|   IBIS file stm32l496_4a6_wlcsp100.ibs
[IBIS ver]   4.2
[File name]   stm32l496_4a6_wlcsp100.ibs
[File Rev]   4.0
[Date]   08-10-2018
[Source]   Data Created at STMicroelectronics
[Notes]   File originated from ELDO simulations.
[Disclaimer]  This information is for modeling purpose only and is
   not guaranteed.
   The information is subject to change without notice.
[Copyright]   Copyright 2018 STMicroelectronics Inc.
|   Component stm32l496_4a6_wlcsp100
[Component] stm32l496_4a6_wlcsp100
[Manufacturer] STMicroelectronics
[Package]
| variable   typ   min   max
R_pkg   0.0   0.0   0.0
L_pkg   0.0H   0.0H   0.0H
C_pkg   0.0F   0.0F   0.0F
[Pin]  signal_name   model_name   R_pin   L_pin   C_pin
A1 VDDUSB POWER
A10 VDD POWER
A2 PA15 io8prog2m25m50m120m_sudq_ft
A3 PD1 io8prog2m25m50m120m_sudq_ft
A4 VDD POWER
A5 PG10 io8prog2m25m50m120m_sudq_ft
A6 VDDIO2 POWER
A7 PB6 io8prog2m25m50m120m_sudq_i2c_ft
A8 PB9 io8prog2m25m50m120m_sudq_i2c_ft
A9 VSS GND
B1 VSS GND
B10 PE3 io8prog2m25m50m120m_sudq_ft
B2 PA14 io8prog2m25m50m120m_sudq_ft
B3 PD0 io8prog2m25m50m120m_sudq_ft
B4 PD4 io8prog2m25m50m120m_sudq_ft
B5 PG9 io8prog2m25m50m120m_sudq_ft
B6 PG12 io8prog2m25m50m120m_sudq_ft
B7 PB5 io8prog2m25m50m120m_sudq_ft
B8 PB8 io8prog2m25m50m120m_sudq_i2c_ft
B9 PE2 io8prog2m25m50m120m_sudq_ft
C1 PA12 io8usblsfs_otg2
C10 VBAT POWER
C2 PA13 io8prog2m25m50m120m_sudq_ft
C3 PC11 io8prog2m25m50m120m_sudq_ft
C4 PC12 io8prog2m25m50m120m_sudq_ft
C5 PD7 io8prog2m25m50m120m_sudq_ft
C6 PB3 io8prog2m25m50m120m_sudq_ft
C7 PB4 io8prog2m25m50m120m_sudq_i2c_ft
C8 PE4 io8prog2m25m50m120m_sudq_ft
C9 PC13 io8prog2m25m50m120m_sudq_ft
D1 PA11 io8usblsfs_otg2
D2 PA10 io8usb_id_otg20_lcd4_ft_ms
D3 PA9 POWER
D4 PC10 io8prog2m25m50m120m_sudq_ft
D5 PD6 io8prog2m25m50m120m_sudq_ft
D6 PG11 io8prog2m25m50m120m_sudq_ft
D7 PB7 io8prog2m25m50m120m_sudq_i2c_ft
D8 PE5 io8prog2m25m50m120m_sudq_ft
D9 VSS GND
D10 PC14-OSC32_IN io8prog2m25m50m120m_sudq_ft
E1 PC8 io8prog2m25m50m120m_sudq_ft
E2 PC9 io8prog2m25m50m120m_sudq_i2c_ft
E3 PA8 io8w_swp_lcd4_ft
E4 PD2 io8prog2m25m50m120m_sudq_ft
E5 PD5 io8prog2m25m50m120m_sudq_ft
E6 PH3-BOOT0 io8prog2m25m50m120m_sudq_ft
E7 PE6 io8prog2m25m50m120m_sudq_ft
E8 NRST ioreset_ft_v33
E9 VDD POWER
E10 PC15-OSC32_OUT io8prog2m25m50m120m_sudq_ft
F1 VDD POWER
F2 PC6 io8prog2m25m50m120m_sudq_ft
F3 PC7 io8prog2m25m50m120m_sudq_ft
F4 PD15 io8prog2m25m50m120m_sudq_ft
F5 PB2 io8prog2m25m50m120m_sudq_ft
F6 PA4 io8prog2m25m50m120m_sudq_ft
F7 PC3 io8prog2m25m50m120m_sudq_ft
F8 PC1 io8prog2m25m50m120m_sudq_i2c_ft
F9 PC0 io8prog2m25m50m120m_sudq_i2c_ft
F10 PH0-OSC_IN io8prog2m25m50m120m_sudq_ft
G1 PD10 io8prog2m25m50m120m_sudq_ft
G10 PH1-OSC_OUT io8prog2m25m50m120m_sudq_ft
G2 PD9 io8prog2m25m50m120m_sudq_ft
G3 PD14 io8prog2m25m50m120m_sudq_ft
G4 PE13 io8prog2m25m50m120m_sudq_ft
G5 PE12 io8prog2m25m50m120m_sudq_ft
G6 PA5 io8prog2m25m50m120m_sudq_ft
G7 VREF+ POWER
G8 VREF- GND
G9 PA0 io8prog2m25m50m120m_sudq_ft
H1 PB15 io8prog2m25m50m120m_sudq_ft
H10 PC2 io8prog2m25m50m120m_sudq_ft
H2 PB14 io8prog2m25m50m120m_sudq_i2c_ft
H3 PD8 io8prog2m25m50m120m_sudq_ft
H4 PE15 io8prog2m25m50m120m_sudq_ft
H5 PE10 io8prog2m25m50m120m_sudq_ft
H6 PC4 io8prog2m25m50m120m_sudq_ft
H7 PA2 io8prog2m25m50m120m_sudq_ft
H8 PA1 io8prog2m25m50m120m_sudq_ft
H9 VSSA GND
J1 PB12 io8w_swp_lcd4_ft
J10 VDDA POWER
J2 PB13 io8prog2m25m50m120m_sudq_i2c_ft
J3 PB11 io8prog2m25m50m120m_sudq_i2c_ft
J4 PE14 io8prog2m25m50m120m_sudq_ft
J5 PE9 io8prog2m25m50m120m_sudq_ft
J6 PB0 io8prog2m25m50m120m_sudq_ft
J7 PA7 io8prog2m25m50m120m_sudq_i2c_ft
J8 VDD POWER
J9 PA3 io8prog2m25m50m120m_sudq_ft
K1 VDD POWER
K10 VSS GND
K2 VSS GND
K3 PB10 io8prog2m25m50m120m_sudq_i2c_ft
K4 PE11 io8prog2m25m50m120m_sudq_ft
K5 PE8 io8prog2m25m50m120m_sudq_ft
K6 PE7 io8prog2m25m50m120m_sudq_ft
K7 PB1 io8prog2m25m50m120m_sudq_ft
K8 PC5 io8prog2m25m50m120m_sudq_ft
K9 PA6 io8prog2m25m50m120m_sudq_ft
[Diff Pin]   inv_pin   vdiff   tdelay_typ  tdelay_min  tdelay_max
C1 D1 200mV   NA   NA   NA
[Model Selector] io8usblsfs_otg2
usb_ls_pd  "USB Low Speed mode - Pull Down"
usb_ls_pu2  "USB Low Speed mode - Pull up 2"
usb_ls_pu  "USB Low Speed mode - Pull up"
usb_fs  "USB Low Speed mode"
usb_fs_pd  "USB Full Speed mode - Pull Down"
usb_fs_pu2  "USB Full Speed mode - Pull up 2"
usb_fs_pu  "USB Full Speed mode - Pull up"
[Model Selector] io8usb_id_otg20_lcd4_ft_ms
io8usbid_1v8_id_pu  "ID 1V8 range with pull up"
io8usbid_3v3_id_pu  "ID 3V3 range with pull up"
io8usbid_1v8_id  "ID 1V8 range"
io8usbid_3v3_id  "ID 3V3 range"
io8lsusbid_1v8_pd  "GPIO 1.8V range with pd io low speed"
io8lsusbid_1v8_pu  "GPIO 1.8V range with pu io low speed"
io8lsusbid_1v8  "GPIO 1.8V range io low speed"
io8lsusbid_3v3_pd  "GPIO 3.3V range with pd io low speed"
io8lsusbid_3v3_pu  "GPIO 3.3V range with pu io low speed"
io8lsusbid_3v3  "GPIO 3.3V range io low speed"
io8fsusbid_1v8_pd  "GPIO 1.8V range with pd io full speed"
io8fsusbid_1v8_pu  "GPIO 1.8V range with pu io full speed"
io8fsusbid_1v8  "GPIO 1.8V range io full speed"
io8fsusbid_3v3_pd  "GPIO 3.3V range with pd io full speed"
io8fsusbid_3v3_pu  "GPIO 3.3V range with pu io full speed"
io8fsusbid_3v3  "GPIO 3.3V range io full speed"
io8msusbid_1v8_pd  "GPIO 1.8V range with pd io medium speed"
io8msusbid_1v8_pu  "GPIO 1.8V range with pu io medium speed"
io8msusbid_1v8  "GPIO 1.8V range io medium speed"
io8msusbid_3v3_pd  "GPIO 3.3V range with pd io medium speed"
io8msusbid_3v3_pu  "GPIO 3.3V range with pu io medium speed"
io8msusbid_3v3  "GPIO 3.3V range io medium speed"
io8hsusbid_1v8_pd  "GPIO 1.8V range with pd io high speed"
io8hsusbid_1v8_pu  "GPIO 1.8V range with pu io high speed"
io8hsusbid_1v8  "GPIO 1.8V range io high speed"
io8hsusbid_3v3_pd  "GPIO 3.3V range with pd io high speed"
io8hsusbid_3v3_pu  "GPIO 3.3V range with pu io high speed"
io8hsusbid_3v3  "GPIO 3.3V range io high speed"
[Model Selector] io8w_swp_lcd4_ft
io8w_swp_classc  "Class C swp functionality"
io8w_swp_classb  "Class B swp functionality"
io8lsw_1v8_pd  "GPIO 1.8V range with pd io low speed"
io8lsw_1v8_pu  "GPIO 1.8V range with pu io low speed"
io8lsw_1v8  "GPIO 1.8V range io low speed"
io8lsw_3v3_pd  "GPIO 3.3V range with pd io low speed"
io8lsw_3v3_pu  "GPIO 3.3V range with pu io low speed"
io8lsw_3v3  "GPIO 3.3V range io low speed"
io8fsw_1v8_pd  "GPIO 1.8V range with pd io full speed"
io8fsw_1v8_pu  "GPIO 1.8V range with pu io full speed"
io8fsw_1v8  "GPIO 1.8V range io full speed"
io8fsw_3v3_pd  "GPIO 3.3V range with pd io full speed"
io8fsw_3v3_pu  "GPIO 3.3V range with pu io full speed"
io8fsw_3v3  "GPIO 3.3V range io full speed"
io8msw_1v8_pd  "GPIO 1.8V range with pd io medium speed"
io8msw_1v8_pu  "GPIO 1.8V range with pu io medium speed"
io8msw_1v8  "GPIO 1.8V range io medium speed"
io8msw_3v3_pd  "GPIO 3.3V range with pd io medium speed"
io8msw_3v3_pu  "GPIO 3.3V range with pu io medium speed"
io8msw_3v3  "GPIO 3.3V range io medium speed"
io8hsw_1v8_pd  "GPIO 1.8V range with pd io high speed"
io8hsw_1v8_pu  "GPIO 1.8V range with pu io high speed"
io8hsw_1v8  "GPIO 1.8V range io high speed"
io8hsw_3v3_pd  "GPIO 3.3V range with pd io high speed"
io8hsw_3v3_pu  "GPIO 3.3V range with pu io high speed"
io8hsw_3v3  "GPIO 3.3V range io high speed"
[Model Selector] io8prog2m25m50m120m_sudq_ft
iols8p_sudq_ft_pd_lv  "IO low speed, PD=40kOhm - 1P8V"
iols8p_sudq_ft_pu_lv  "IO low speed, PU=40kOhm - 1P8V"
iols8p_sudq_ft_lv  "IO low speed - 1P8V"
iols8p_sudq_ft_pd  "IO low speed, PD=40kOhm - 3P3V"
iols8p_sudq_ft_pu  "IO low speed, PU=40kOhm - 3P3V"
iols8p_sudq_ft  "IO low speed - 3P3V"
iofs8p_sudq_ft_pd_lv  "IO full speed, PD=40kOhm - 1P8V"
iofs8p_sudq_ft_pu_lv  "IO full speed, PU=40kOhm - 1P8V"
iofs8p_sudq_ft_lv  "IO full speed - 1P8V"
iofs8p_sudq_ft_pd  "IO full speed, PD=40kOhm - 3P3V"
iofs8p_sudq_ft_pu  "IO full speed, PU=40kOhm - 3P3V"
iofs8p_sudq_ft  "IO full speed - 3P3V"
ioms8p_sudq_ft_pd_lv  "IO medium speed, PD=40kOhm - 1P8V"
ioms8p_sudq_ft_pu_lv  "IO medium speed, PU=40kOhm - 1P8V"
ioms8p_sudq_ft_lv  "IO medium speed - 1P8V"
ioms8p_sudq_ft_pd  "IO medium speed, PD=40kOhm - 3P3V"
ioms8p_sudq_ft_pu  "IO medium speed, PU=40kOhm - 3P3V"
ioms8p_sudq_ft  "IO medium speed - 3P3V"
iohs8p_sudq_ft_pd_lv  "IO high speed, PD=40kOhm - 1P8V"
iohs8p_sudq_ft_pu_lv  "IO high speed, PU=40kOhm - 1P8V"
iohs8p_sudq_ft_lv  "IO high speed - 1P8V"
iohs8p_sudq_ft_pd  "IO high speed, PD=40kOhm - 3P3V"
iohs8p_sudq_ft_pu  "IO high speed, PU=40kOhm - 3P3V"
iohs8p_sudq_ft  "IO high speed - 3P3V"
[Model Selector] io8prog2m25m50m120m_sudq_i2c_ft
io8prog_1v8_i2c_pd  "5V Tol GPIO 1.8V range i2c functionality with pull down"
io8prog_1v8_i2c_pu  "5V Tol GPIO 1.8V range i2c functionality with pull up"
io8prog_1v8_i2c  "5V Tol GPIO 1.8V range i2c functionality"
io8prog_3v3_i2c_pd  "5V Tol GPIO 3.3V range i2c functionality with pull down"
io8prog_3v3_i2c_pu  "5V Tol GPIO 3.3V range i2c functionality with pull up"
io8prog_3v3_i2c  "5V Tol GPIO 3.3V range i2c functionality"
io8ls_1v8_pd  "5V Tol GPIO 1.8V range with pd io low speed"
io8ls_1v8_pu  "5V Tol GPIO 1.8V range with pu io low speed"
io8ls_1v8  "5V Tol GPIO 1.8V range io low speed"
io8ls_3v3_pd  "5V Tol GPIO 3.3V range with pd io low speed"
io8ls_3v3_pu  "5V Tol GPIO 3.3V range with pu io low speed"
io8ls_3v3  "5V Tol GPIO 3.3V range io low speed"
io8fs_1v8_pd  "5V Tol GPIO 1.8V range with pd io full speed"
io8fs_1v8_pu  "5V Tol GPIO 1.8V range with pu io full speed"
io8fs_1v8  "5V Tol GPIO 1.8V range io full speed"
io8fs_3v3_pd  "5V Tol GPIO 3.3V range with pd io full speed"
io8fs_3v3_pu  "5V Tol GPIO 3.3V range with pu io full speed"
io8fs_3v3  "5V Tol GPIO 3.3V range io full speed"
io8ms_1v8_pd  "5V Tol GPIO 1.8V range with pd io medium speed"
io8ms_1v8_pu  "5V Tol GPIO 1.8V range with pu io medium speed"
io8ms_1v8  "5V Tol GPIO 1.8V range io medium speed"
io8ms_3v3_pd  "5V Tol GPIO 3.3V range with pd io medium speed"
io8ms_3v3_pu  "5V Tol GPIO 3.3V range with pu io medium speed"
io8ms_3v3  "5V Tol GPIO 3.3V range io medium speed"
io8hs_1v8_pd  "5V Tol GPIO 1.8V range with pd io high speed"
io8hs_1v8_pu  "5V Tol GPIO 1.8V range with pu io high speed"
io8hs_1v8  "5V Tol GPIO 1.8V range io high speed"
io8hs_3v3_pd  "5V Tol GPIO 3.3V range with pd io high speed"
io8hs_3v3_pu  "5V Tol GPIO 3.3V range with pu io high speed"
io8hs_3v3  "5V Tol GPIO 3.3V range io high speed"
[Model Selector] ioreset_ft_v33
ioreset_1v2_pu  "RESET 1.2V range with PU"
ioreset_1v2  "RESET 1.2V range"
ioreset_1v8_pu  "RESET 1.8V range with PU"
ioreset_1v8  "RESET 1.8V range"
ioreset_3v3_pu  "RESET 3.3V range with PU"
ioreset_3v3  "RESET 3.3V range"
| Models and submodels in the file (121): usb_ls_pd (I/O), usb_ls_pu2 (I/O), usb_ls_pu (I/O), usb_fs (I/O), usb_fs_pd (I/O), usb_fs_pu2 (I/O), usb_fs_pu (I/O), io8usbid_1v8_id_pu (Input), io8usbid_3v3_id_pu (Input), io8usbid_1v8_id (Input), io8usbid_3v3_id (Input), io8lsusbid_1v8_pd (I/O), io8lsusbid_1v8_pu (I/O), io8lsusbid_1v8 (I/O), io8lsusbid_3v3_pd (I/O), io8lsusbid_3v3_pu (I/O), io8lsusbid_3v3 (I/O), io8fsusbid_1v8_pd (I/O), io8fsusbid_1v8_pu (I/O), io8fsusbid_1v8 (I/O), io8fsusbid_3v3_pd (I/O), io8fsusbid_3v3_pu (I/O), io8fsusbid_3v3 (I/O), io8msusbid_1v8_pd (I/O), io8msusbid_1v8_pu (I/O), io8msusbid_1v8 (I/O), io8msusbid_3v3_pd (I/O), io8msusbid_3v3_pu (I/O), io8msusbid_3v3 (I/O), io8hsusbid_1v8_pd (I/O), io8hsusbid_1v8_pu (I/O), io8hsusbid_1v8 (I/O), io8hsusbid_3v3_pd (I/O), io8hsusbid_3v3_pu (I/O), io8hsusbid_3v3 (I/O), io8w_swp_classc (I/O), io8w_swp_classb (I/O), io8lsw_1v8_pd (I/O), io8lsw_1v8_pu (I/O), io8lsw_1v8 (I/O), io8lsw_3v3_pd (I/O), io8lsw_3v3_pu (I/O), io8lsw_3v3 (I/O), io8fsw_1v8_pd (I/O), io8fsw_1v8_pu (I/O), io8fsw_1v8 (I/O), io8fsw_3v3_pd (I/O), io8fsw_3v3_pu (I/O), io8fsw_3v3 (I/O), io8msw_1v8_pd (I/O), io8msw_1v8_pu (I/O), io8msw_1v8 (I/O), io8msw_3v3_pd (I/O), io8msw_3v3_pu (I/O), io8msw_3v3 (I/O), io8hsw_1v8_pd (I/O), io8hsw_1v8_pu (I/O), io8hsw_1v8 (I/O), io8hsw_3v3_pd (I/O), io8hsw_3v3_pu (I/O), io8hsw_3v3 (I/O), iols8p_sudq_ft_pd_lv (I/O), iols8p_sudq_ft_pu_lv (I/O), iols8p_sudq_ft_lv (I/O), iols8p_sudq_ft_pd (I/O), iols8p_sudq_ft_pu (I/O), iols8p_sudq_ft (I/O), iofs8p_sudq_ft_pd_lv (I/O), iofs8p_sudq_ft_pu_lv (I/O), iofs8p_sudq_ft_lv (I/O), iofs8p_sudq_ft_pd (I/O), iofs8p_sudq_ft_pu (I/O), iofs8p_sudq_ft (I/O), ioms8p_sudq_ft_pd_lv (I/O), ioms8p_sudq_ft_pu_lv (I/O), ioms8p_sudq_ft_lv (I/O), ioms8p_sudq_ft_pd (I/O), ioms8p_sudq_ft_pu (I/O), ioms8p_sudq_ft (I/O), iohs8p_sudq_ft_pd_lv (I/O)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
